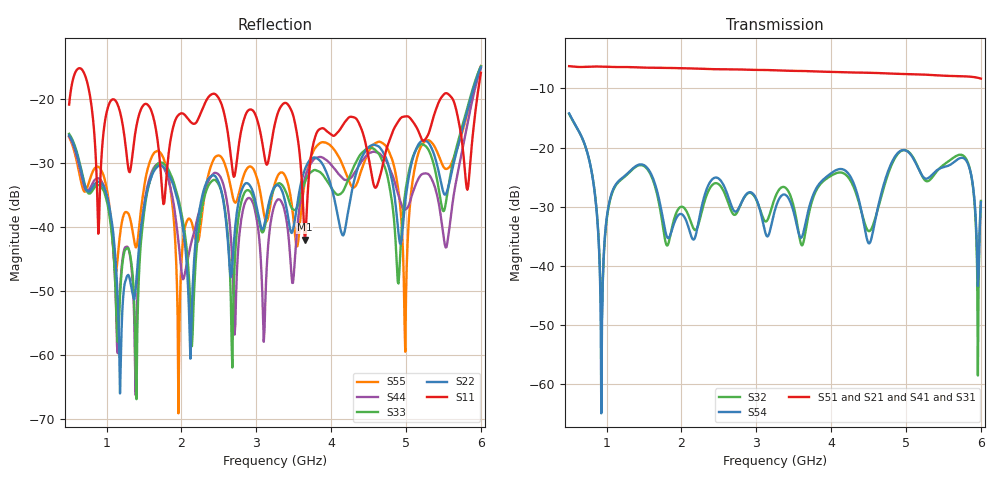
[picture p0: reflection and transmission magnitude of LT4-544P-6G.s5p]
! MTS Systemtechnik GmbH
! S-Parameters
! Model: LT4-544P-6G
! Rohde & Schwarz ZVB8 2Ports - Version 3.20 - 1145.1010k08 SN: 100119
! Converted & adapted with MATLAB
!		|  MTS  |
!		|  |--o OUT 4 (Port 5)
!		|  |--o OUT 3 (Port 4)
! C (Port 1) o--| LT4-544P-6G |
!		|  |--o OUT 2 (Port 3)
!		|  |--o OUT 1 (Port 2)
! S5P File: Measurements:
! <S11,S12,S13,S14,S15>,
! <S21,S22,S23,S24,S25>,
! <S31,S32,S33,S34,S35>,
! <S41,S42,S43,S44,S45>,
! <S51,S52,S53,S54,S55>:
# HZ  S  DB  R  50.00
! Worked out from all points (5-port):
!   551 points, 500 MHz to 6 GHz, reference 50 ohm
!   strongest paths, dB at 500 MHz, 1.87 GHz, 3.25 GHz, 4.63 GHz, 6 GHz:
!     S51: -6.2, -6.5, -6.9, -7.4, -8.3
!     S21: -6.2, -6.5, -6.9, -7.4, -8.3
!     S41: -6.2, -6.5, -6.9, -7.4, -8.3
!     S31: -6.2, -6.5, -7.0, -7.4, -8.4
!     S54: -14.2, -34.1, -30.5, -29.8, -29.2
!     S32: -14.3, -33.8, -28.5, -30.1, -29.0
!   lowest |S11| = -42.0 dB at 3.65 GHz (marker M1), VSWR 1.02, Z = 50.1 + j0.781 ohm
!   |S11| at or under -10 dB: start of sweep to end of sweep
